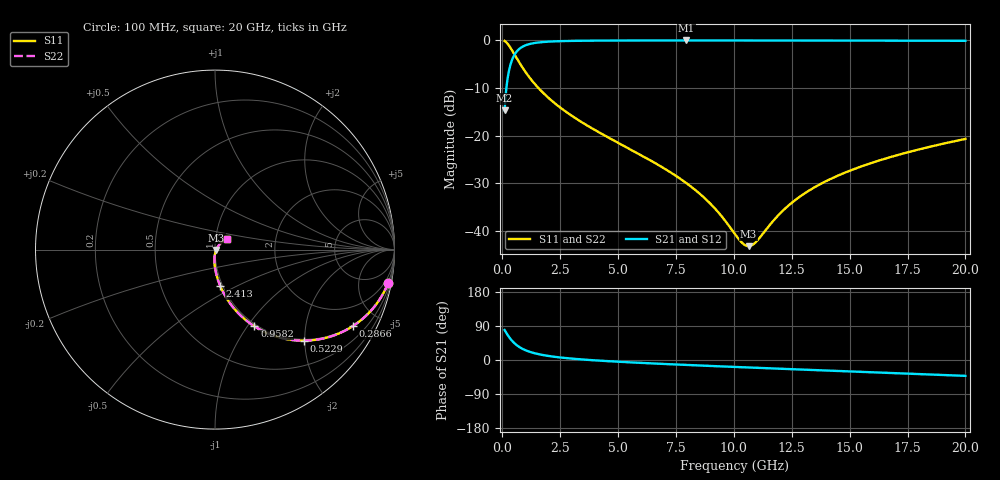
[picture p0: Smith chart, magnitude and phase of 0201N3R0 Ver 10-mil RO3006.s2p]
# GHz S MA R 50
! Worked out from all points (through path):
!   1601 points, 100 MHz to 20 GHz, reference 50 ohm
!   highest |S21| = -0.06 dB at 7.948 GHz (marker M1); lowest = -14.6 dB at 100 MHz (marker M2)
!   group delay of S21, straight-line fit = 9.13 ps
!   lowest |S11| = -43.1 dB at 10.63 GHz (marker M3), VSWR 1.01, Z = 50.7 - j0.261 ohm
!   |S11| at or under -10 dB: 1.557 GHz to end of sweep
!   |S22| runs from -43.1 to -0.2 dB; largest |S21 - S12| = 0
!   S11 on the Smith chart (normalised r, x): 100 MHz: 1, -10; 286.6 MHz: 0.97, -3.64; 522.9 MHz: 0.97, -1.99; 958.2 MHz: 0.97, -1.08; 2.413 GHz: 0.97, -0.41; 20 GHz: 1.14, +0.14
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0.1  0.9826 -10.9  0.1853 79.1  0.1853 79.1  0.9826 -10.9
0.1870625  0.9428 -19.8  0.3326 70.2  0.3326 70.2  0.9428 -19.8
0.2865625  0.8792 -28.9  0.4753 61.0  0.4753 61.0  0.8792 -28.9
0.3985  0.7985 -37.7  0.6006 52.2  0.6006 52.2  0.7985 -37.7
0.522875  0.7106 -45.6  0.702 44.3  0.702 44.3  0.7106 -45.6
0.721875  0.5897 -55.0  0.8057 34.8  0.8057 34.8  0.5897 -55.0
0.9581875  0.4808 -62.8  0.8747 26.9  0.8747 26.9  0.4808 -62.8
1.505437  0.3263 -73.3  0.9427 16.2  0.9427 16.2  0.3263 -73.3
2.413375  0.2047 -81.8  0.9755 7.3  0.9755 7.3  0.2047 -81.8
3.420812  0.1389 -86.8  0.9864 1.6  0.9864 1.6  0.1389 -86.8
6.741625  0.04936 -93.4  0.9932 -9.8  0.9932 -9.8  0.04936 -93.4
7.948062  0.03188 -92.3  0.9933 -13.0  0.9933 -13.0  0.03188 -92.3
9.067438  0.01852 -85.7  0.9932 -15.9  0.9932 -15.9  0.01852 -85.7
10.05  0.009302 -61.8  0.993 -18.4  0.993 -18.4  0.009302 -61.8
10.38581  0.007433 -41.6  0.9929 -19.2  0.9929 -19.2  0.007433 -41.6
10.63456  0.006966 -21.7  0.9928 -19.8  0.9928 -19.8  0.006966 -21.7
10.97038  0.007772 3.8  0.9926 -20.6  0.9926 -20.6  0.007772 3.8
12.26388  0.01769 41.1  0.992 -23.7  0.992 -23.7  0.01769 41.1
13.37081  0.02776 47.1  0.9914 -26.3  0.9914 -26.3  0.02776 47.1
14.826  0.04127 48.5  0.9904 -29.7  0.9904 -29.7  0.04127 48.5
16.69162  0.05899 47.1  0.9889 -34.1  0.9889 -34.1  0.05899 47.1
20  0.09247 41.9  0.9852 -41.9  0.9852 -41.9  0.09247 41.9
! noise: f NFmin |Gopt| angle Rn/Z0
0.1  0.0009587  0.9553  0.5096  0.004834
2.301  0.005387  0.8267  4.548  0.006529
4.515  0.008895  0.7977  8.605  0.009051
6.729  0.01202  0.7797  12.67  0.01104
8.943  0.01491  0.7667  16.72  0.01273
11.14  0.01764  0.7568  20.71  0.01421
13.36  0.02028  0.7491  24.69  0.01555
15.57  0.02286  0.7431  28.62  0.01679
17.79  0.02539  0.7384  32.5  0.01794
20  0.02789  0.7349  36.32  0.01902
